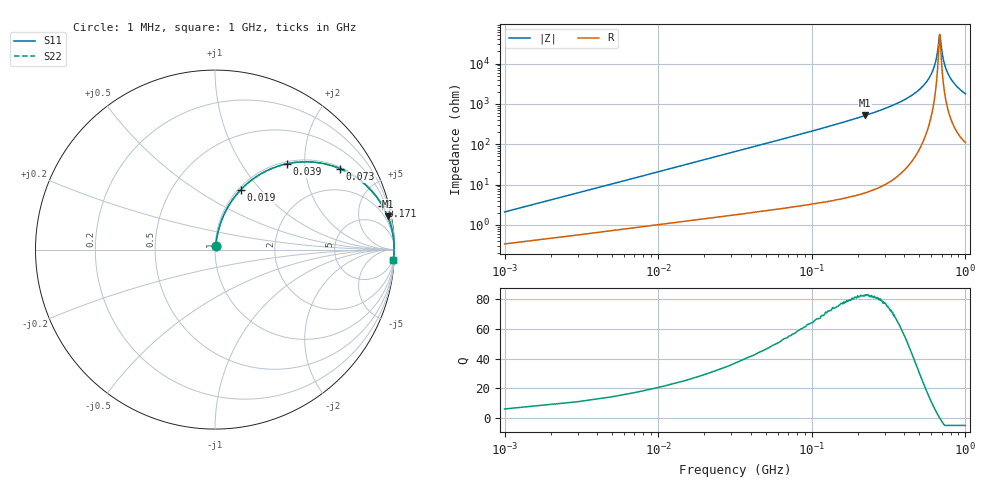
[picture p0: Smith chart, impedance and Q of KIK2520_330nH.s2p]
!version-2
!date-01.2022
!Series
# MHz S RI R 50
!Freq ReS11 ImS11 ReS21 ImS21 ReS12 ImS12 ReS22 ImS22
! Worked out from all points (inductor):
!   501 points, 1 MHz to 1 GHz, reference 50 ohm
!   read as one part in series: L = 330 nH near 5 MHz
!   highest Q = 82.8 at 223 MHz (marker M1), where L = 370 nH
!   self-resonance near 679 MHz
!   S11 on the Smith chart (normalised r, x): 1 MHz: 1.01, +0.04; 19 MHz: 1.03, +0.79; 39 MHz: 1.04, +1.62; 73 MHz: 1.06, +3.06; 171 MHz: 1.10, +7.57; 1 GHz: 3, -36
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1  0.00379 0.0206  0.9962 -0.0206  0.9962 -0.0206  0.00379 0.0206
9  0.0422 0.1771  0.9578 -0.1771  0.9578 -0.1771  0.0422 0.1771
19  0.1432 0.3332  0.8568 -0.3332  0.8568 -0.3332  0.1432 0.3332
39  0.3995 0.4778  0.6005 -0.4778  0.6005 -0.4778  0.3995 0.4778
73  0.6978 0.4503  0.3022 -0.4503  0.3022 -0.4503  0.6978 0.4503
111  0.8446 0.3549  0.1554 -0.3549  0.1554 -0.3549  0.8446 0.3549
169  0.9304 0.2483  0.0696 -0.2483  0.0696 -0.2483  0.9304 0.2483
171  0.932 0.2454  0.068 -0.2454  0.068 -0.2454  0.932 0.2454
223  0.962 0.1853  0.038 -0.1853  0.038 -0.1853  0.962 0.1853
335  0.9868 0.1075  0.0132 -0.1075  0.0132 -0.1075  0.9868 0.1075
501  0.9966 0.0439  0.00338 -0.0439  0.00338 -0.0439  0.9966 0.0439
565  0.9977 0.0265  0.00226 -0.0265  0.00226 -0.0265  0.9977 0.0265
613  0.9981 0.0148  0.0019 -0.0148  0.0019 -0.0148  0.9981 0.0148
645  0.9982 0.00764  0.00183 -0.00764  0.00183 -0.00764  0.9982 0.00764
667  0.9982 0.0029  0.00185 -0.0029  0.00185 -0.0029  0.9982 0.0029
677  0.9981 0.000801  0.00187 -0.000801  0.00187 -0.000801  0.9981 0.000801
683  0.9981 -0.000444  0.0019 0.000444  0.0019 0.000444  0.9981 -0.000444
707  0.998 -0.00532  0.00201 0.00532  0.00201 0.00532  0.998 -0.00532
735  0.9978 -0.0108  0.00221 0.0108  0.00221 0.0108  0.9978 -0.0108
777  0.9974 -0.0187  0.00261 0.0187  0.00261 0.0187  0.9974 -0.0187
835  0.9966 -0.0289  0.00337 0.0289  0.00337 0.0289  0.9966 -0.0289
1000  0.9935 -0.0552  0.00649 0.0552  0.00649 0.0552  0.9935 -0.0552
